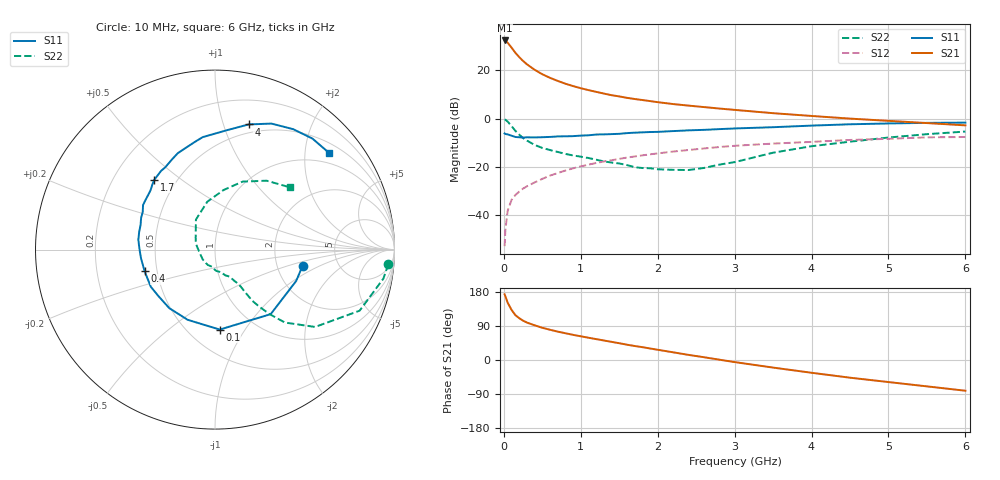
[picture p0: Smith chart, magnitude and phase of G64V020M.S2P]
! SIEMENS Small Signal Semiconductors
! BFG193
! Si NPN RF Bipolar Junction Transistor in SOT223
! VCE = 4 V  IC = 20 mA
! Common Emitter S-Parameters:  August  1996
# GHz  S  MA  R  50
!  f  S11  S21  S12  S22
! GHz  MAG  ANG  MAG  ANG  MAG  ANG  MAG  ANG
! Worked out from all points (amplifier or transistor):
!   36 points, 10 MHz to 6 GHz, reference 50 ohm
!   highest |S21| = 32.4 dB at 10 MHz (marker M1)
!   |S21| within 3 dB of that: start of sweep to 101 MHz
!   unconditionally stable (mu >= 1): 709.2 MHz to 2.472 GHz
!   at 250 MHz: K = 0.74, MSG = 26.4 dB, |S12| = -28.9 dB
!   at 1.4 GHz: K = 1.05, MAG = 12.1 dB, |S12| = -17.2 dB
!   at 6 GHz: K = 0.88, MSG = 2.4 dB, |S12| = -7.6 dB
!   S11 on the Smith chart (normalised r, x): 10 MHz: 2.79, -0.66; 100 MHz: 0.70, -0.78; 400 MHz: 0.43, -0.12; 1.7 GHz: 0.38, +0.40; 4 GHz: 0.42, +1.22; 6 GHz: 0.72, +2.55
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0.01  0.4964 -10.4  41.88 173.4  0.0023 90.8  0.9692 -4.8
0.02  0.4849 -21.1  41.27 168.1  0.005 81.3  0.9519 -9.8
0.05  0.475 -49.2  37.56 151.1  0.0125 72.3  0.8747 -22.9
0.1  0.4463 -86.6  29.8 132.3  0.0209 64.7  0.7048 -37.7
0.15  0.4198 -111.3  23.27 118.4  0.0264 59.3  0.5631 -46.2
0.2  0.4139 -128.0  18.95 110.3  0.031 59.0  0.4702 -49.8
0.25  0.408 -140.7  15.75 103.8  0.0358 58.7  0.3983 -52.3
0.3  0.4132 -149.9  13.44 98.8  0.0399 59.3  0.3537 -53.9
0.4  0.4104 -162.8  10.36 91.6  0.048 60.5  0.2877 -54.8
0.5  0.4152 -173.5  8.36 85.0  0.057 60.2  0.2492 -55.2
0.6  0.421 179.4  7.048 79.8  0.0665 60.4  0.2252 -56.3
0.7  0.4307 172.6  6.088 74.9  0.0752 60.2  0.2057 -58.2
0.9  0.4368 161.7  4.757 66.4  0.0942 58.0  0.174 -60.9
1.1  0.4542 152.4  3.921 58.8  0.1121 55.6  0.1541 -68.4
1.4  0.4812 140.6  3.081 47.9  0.1383 50.2  0.124 -80.6
1.7  0.5156 130.9  2.568 37.0  0.1657 44.9  0.0997 -96.5
2.2  0.5558 115.7  2.018 20.3  0.2094 34.0  0.0876 -141.2
3.5  0.6689 84.2  1.306 -20.0  0.3066 4.2  0.1983 122.4
4  0.7219 75.0  1.144 -33.7  0.3323 -5.5  0.2703 99.1
4.5  0.7692 65.9  1.008 -46.7  0.3643 -15.6  0.3355 81.8
5.5  0.8231 48.7  0.815 -69.6  0.4127 -39.2  0.48 53.1
6  0.833 40.3  0.731 -81.1  0.4192 -52.7  0.5441 39.5
